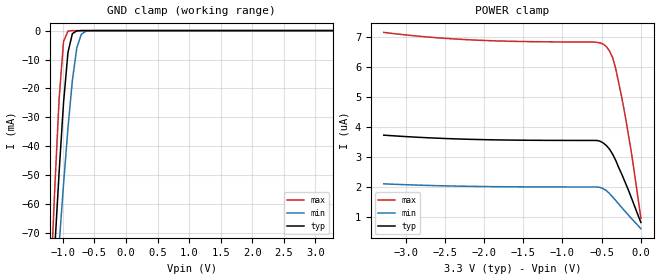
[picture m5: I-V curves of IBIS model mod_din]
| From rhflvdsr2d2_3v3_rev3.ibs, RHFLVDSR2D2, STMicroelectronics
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|   Model mod_din
[Model]   mod_din
Model_type Input
Vinl   =   0.8000V
Vinh   =   2.0000V
C_comp   0.075pF   0.072pF   0.079pF
[Temperature Range]  25.0000   0.1250k   -55.0000
[Voltage Range]   3.3000V   3.0000V   3.6000V
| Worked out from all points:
|   GND clamp passes 1 mA (typ) near -0.85 V on its own axis
[GND_clamp]
|Voltage   I(typ)   I(min)   I(max)
-3.3V     -1.037A    -847.3mA   -1.291A
-1.2V     -103.9mA   -118.4mA   -90.61mA
-1.13V    -75.7mA    -95.97mA   -55.15mA
-1.06V    -48.92mA   -74.09mA   -23.64mA
-990mV    -24.98mA   -53.14mA   -3.768mA
-920mV    -7.585mA   -33.75mA   -179.6uA
-850mV    -1.057mA   -17.22mA   -5.053uA
-780mV    -97.1uA    -5.969mA   -122.7nA
-710mV    -6.82uA    -1.339mA   -2.974nA
-640mV    -449.9nA   -233.7uA   -80.51pA
-500mV    -1.943nA   -4.459uA   -7.043pA
3.28V     3.538uA    1.987uA    6.819uA
[POWER_clamp]
|Voltage   I(typ)   I(min)   I(max)
-3.28V    3.717uA    2.092uA    7.145uA
-2.24V    3.582uA    2.011uA    6.906uA
-560mV    3.539uA    1.988uA    6.813uA
-480mV    3.455uA    1.928uA    6.753uA
-440mV    3.369uA    1.867uA    6.673uA
-400mV    3.249uA    1.766uA    6.522uA
-360mV    3.079uA    1.654uA    6.302uA
-320mV    2.869uA    1.533uA    5.922uA
-240mV    2.389uA    1.289uA    4.922uA
-200mV    2.138uA    1.169uA    4.362uA
-120mV    1.618uA    937nA      3.121uA
0V        803nA      596.8nA    940.7nA
